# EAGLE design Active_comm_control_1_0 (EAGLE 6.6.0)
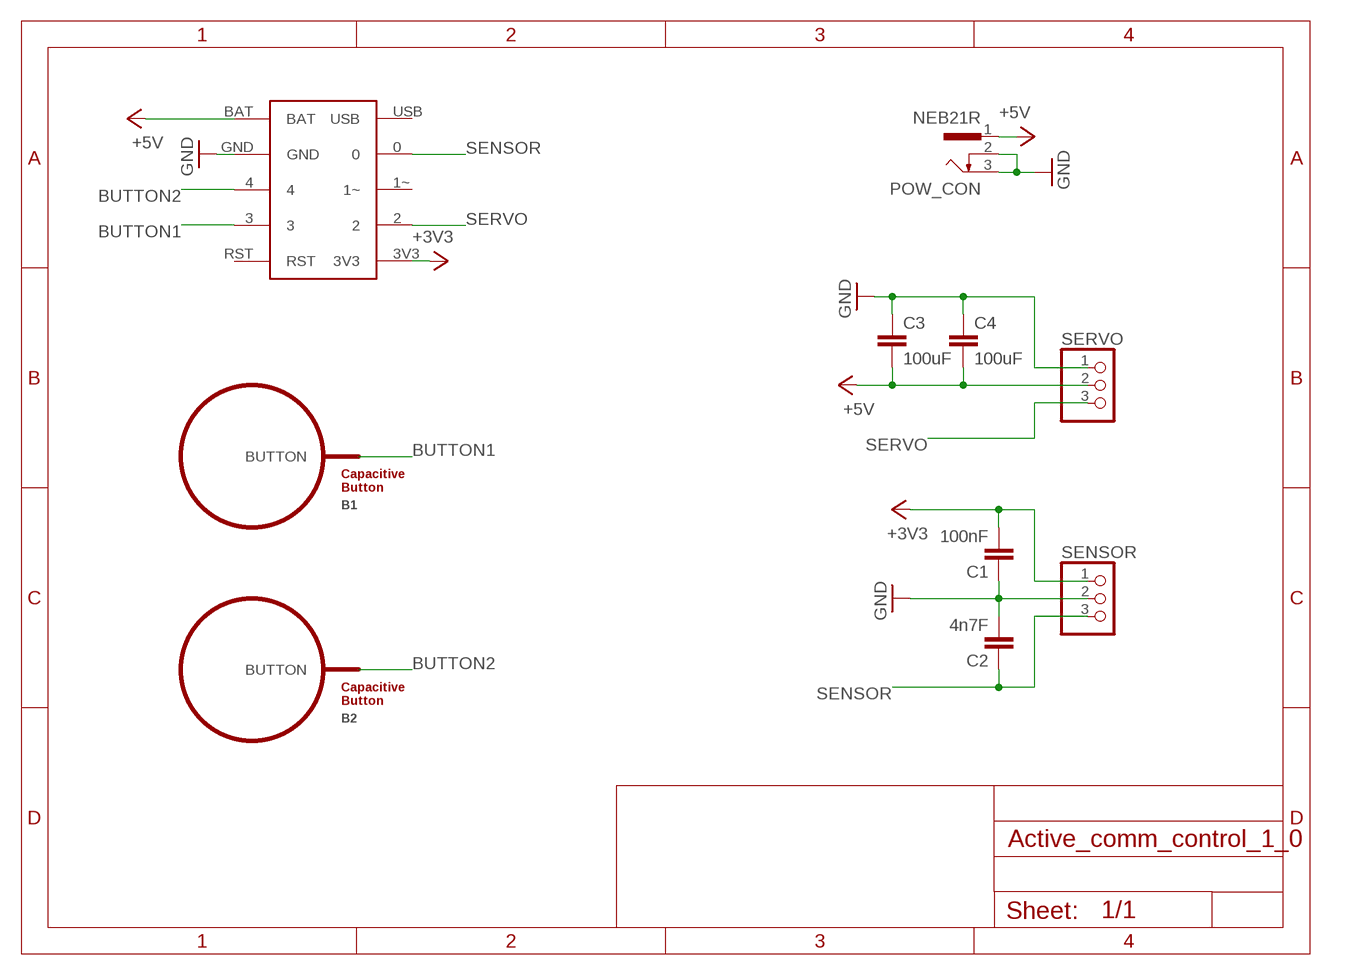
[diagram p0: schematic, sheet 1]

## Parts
B1  BUTTON_PASSIVE10MM  [BUTTON_PASSIVE_10MM]
B2  BUTTON_PASSIVE10MM  [BUTTON_PASSIVE_10MM]
C1  100nF  C-EUC0805  [C0805]
C2  4n7F  C-EUC0805  [C0805]
C3  100uF  C-EUC1206  [C1206]
C4  100uF  C-EUC1206  [C1206]
POW_CON  NEB21R  [NEB21R]
SENSOR  PINHD-1X3  [1X03]
SERVO  PINHD-1X3  [1X03]
TRINKET-M0  TRINKET-M0  [TRINKET-M0-NO-HOLES]

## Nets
+3V3: C1.2 SENSOR.1 TRINKET-M0.3V3
+5V: C3.2 C4.2 POW_CON.1 SERVO.2 TRINKET-M0.BAT
BUTTON1: B1.BUTTON TRINKET-M0.3
BUTTON2: B2.BUTTON TRINKET-M0.4
GND: C1.1 C2.2 C3.1 C4.1 POW_CON.2 POW_CON.3 SENSOR.2 SERVO.1 TRINKET-M0.GND
SENSOR: C2.1 SENSOR.3 TRINKET-M0.0
SERVO: SERVO.3 TRINKET-M0.2
Unconnected: TRINKET-M0.1~ TRINKET-M0.RST TRINKET-M0.USB

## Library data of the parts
B1 B2 = TouchWidgets:BUTTON_PASSIVE: Button, Passive Capacitive/Touch Sensing Type
C1 C2 = resistor:C-EU: CAPACITOR, European symbol
C3 C4 = rcl:C-EU: CAPACITOR, European symbol
POW_CON = con-lumberg:NEB21R: Netzgeräte-Einbaukupplung abgewinkelte Ausführung mit Öffner Source: http://www.lumberg.com/Produkte/PDFs/NEB21R.pdf; MPN: NEB 21 R; OC_FARNELL: 1217037; OC_NEWARK: 97K6458
SENSOR SERVO = adafruit:PINHD-1X3: PIN HEADER
TRINKET-M0 = adafruit:TRINKET-M0

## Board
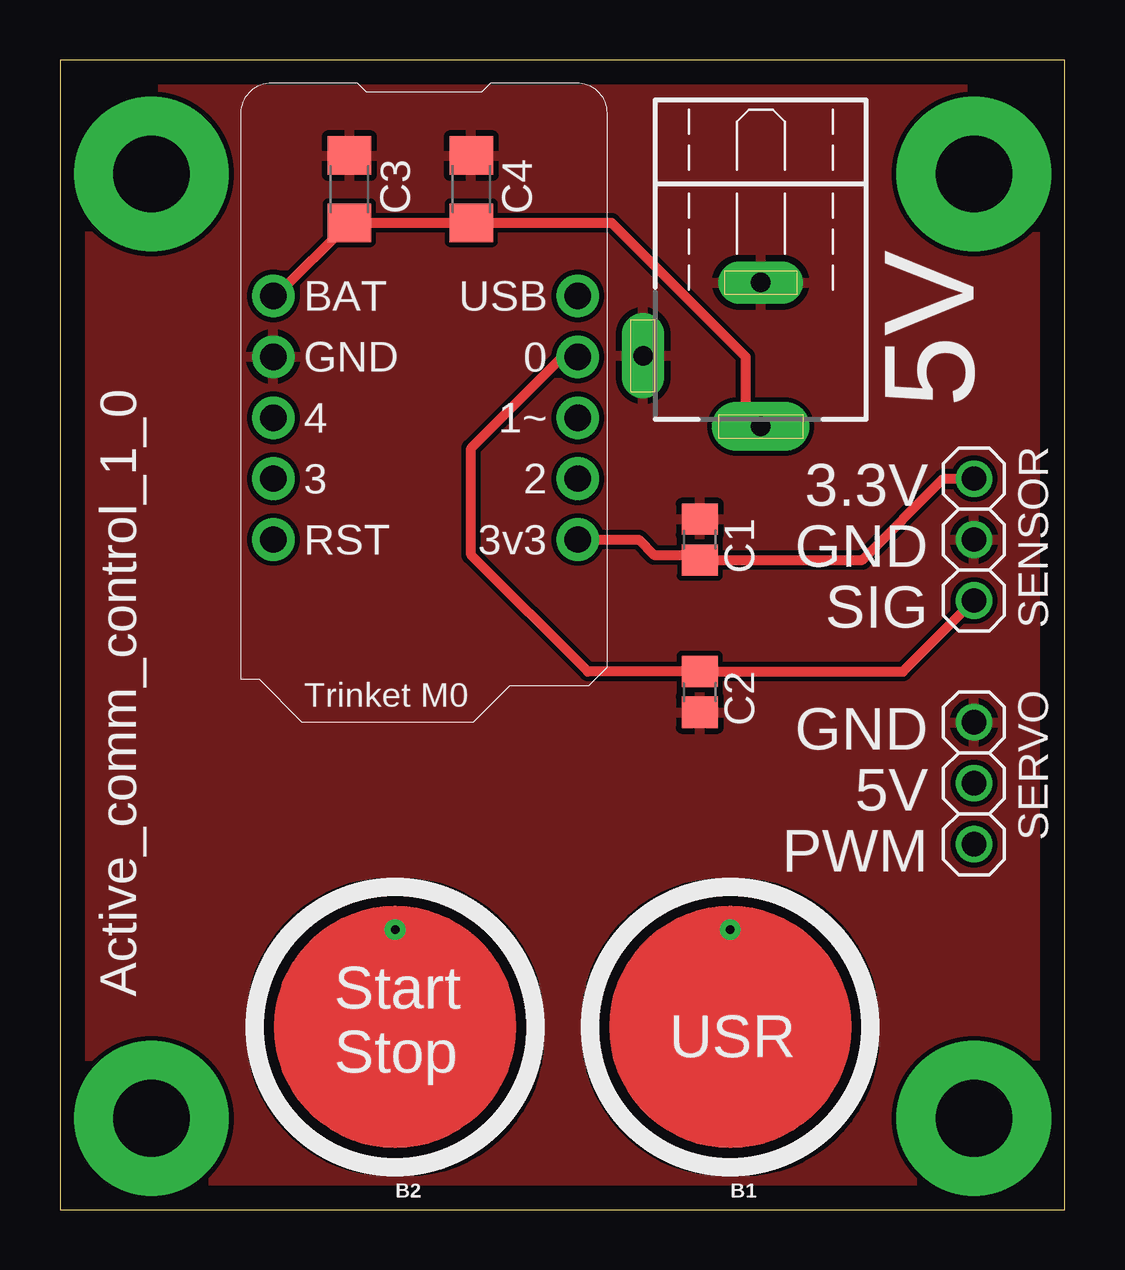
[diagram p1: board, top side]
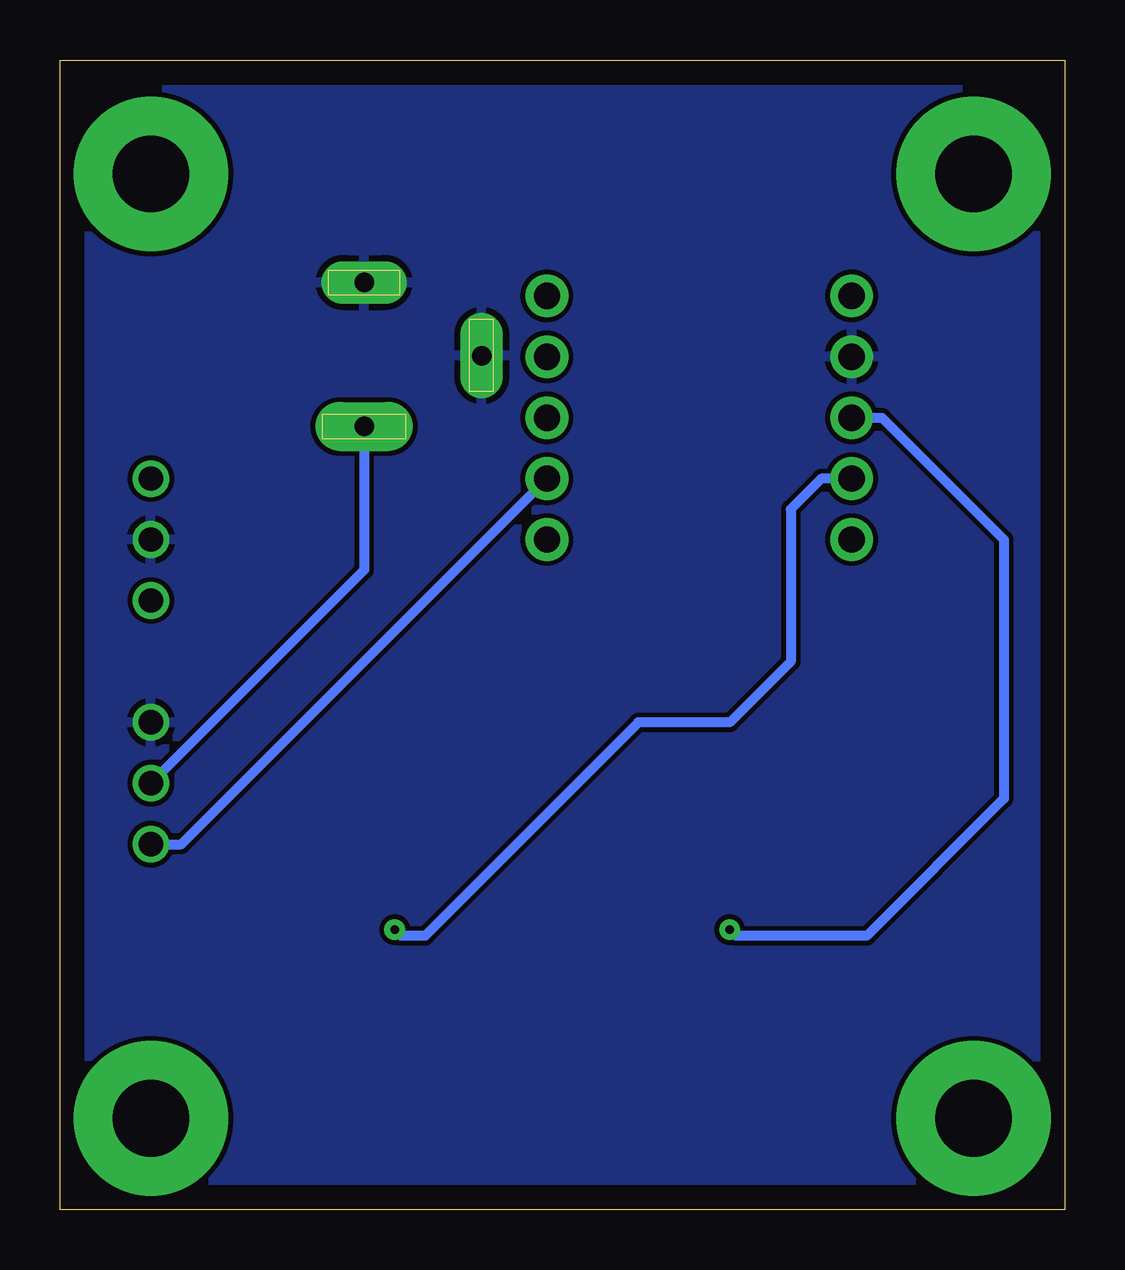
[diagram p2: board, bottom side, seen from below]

Size 41.89 x 47.93 mm. Coordinates in mm from the lower left corner, seen from the top.
Outline: 0,0 41.89,0 41.89,47.93 0,47.93 0,0
Copper layers (1*16): Top 0.035mm / dielectric 1.5mm / Bottom 0.035mm
Design rules "default": minimum track width 10mil, minimum drill 24mil, track to track 8mil, track to pad 8mil, pad to pad 8mil, via to via 8mil, smd to smd 8mil, copper to edge 40mil, drill to drill 8mil, minimum pad ring 10mil, minimum via ring 8mil, stop-mask expansion 4mil, vias tented up to drill 0mil, thermal gap 10mil

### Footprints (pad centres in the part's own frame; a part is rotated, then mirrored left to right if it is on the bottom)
BUTTON_PASSIVE_10MM = drill 0.356: BUTTON 0,4.064
C0805 = smd 1.3 x 1.5: 1 -0.85,0; 2 0.85,0
C1206 = smd 1.6 x 1.8: 1 -1.4,0; 2 1.4,0
NEB21R = drill 0.813 pad 2.032 long: 1 0,7.35 | drill 0.813 pad 1.778 long: 2 4.9,4.4; 3 0,1.35
1X03 = drill 1.016: 1 -2.54,0; 2 0,0; 3 2.54,0
TRINKET-M0-NO-HOLES = drill 1.1 pad 1.778: 0 6.35,2.54; 1~ 6.35,0; 2 6.35,-2.54; 3 -6.35,-2.54; 3V3 6.35,-5.08; 4 -6.35,0; BAT -6.35,5.08; GND -6.35,2.54; RST -6.35,-5.08; USB 6.35,5.08

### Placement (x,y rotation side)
B1  27.94,7.62 0 top
B2  13.97,7.62 0 top
C1  26.67,27.94 270 top
C2  26.67,21.59 270 top
C3  12.06,42.55 270 top
C4  17.14,42.55 270 top
POW_CON  29.21,40.01 180 top
SENSOR  38.1,27.94 270 top
SERVO  38.1,17.78 270 top
TRINKET-M0  15.24,33.02 0 top

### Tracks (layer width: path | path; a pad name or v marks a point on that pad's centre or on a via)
+3V3
  Top 0.406: TRINKET-M0.3V3 24.13,27.94 24.77,27.3 26.45,27.3 C1.2 33.44,27.09 36.83,30.48 SENSOR.1
+5V
  Top 0.406: TRINKET-M0.BAT 9.02,38.1 C3.2 C4.2 22.99,41.15 28.57,35.56 28.57,33.29 POW_CON.1
  Bottom 0.406: POW_CON.1 29.21,26.67 SERVO.2
BUTTON1
  Bottom 0.406: TRINKET-M0.3 10.16,30.48 11.43,29.21 11.43,22.86 13.97,20.32 17.78,20.32 26.67,11.43 27.69,11.43 B1.BUTTON
BUTTON2
  Bottom 0.406: TRINKET-M0.4 7.62,33.02 2.54,27.94 2.54,17.14 8.26,11.43 13.72,11.43 B2.BUTTON
GND
  pour Bottom: 0,48.26 0,0 41.91,0 41.91,48.26
  pour Top: 0,48.26 0,0 41.91,0 41.91,48.26
N$1  (via drill 3.2 pad 6.45)
  other vias: 38.1,3.81
N$2  (via drill 3.2 pad 6.45)
  other vias: 38.1,43.18
N$3  (via drill 3.2 pad 6.45)
  other vias: 3.81,43.18
N$4  (via drill 3.2 pad 6.45)
  other vias: 3.81,3.81
SENSOR
  Top 0.406: SENSOR.3 35.14,22.44 C2.1 22.01,22.44 17.14,27.3 17.14,31.75 20.95,35.56 TRINKET-M0.0
SERVO
  Bottom 0.406: SERVO.3 36.83,15.24 TRINKET-M0.2

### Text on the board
tPlace: 5V | 3.3V | GND | SIG | GND | 5V | PWM | Active_comm_control_1_0 | Start / Stop | USR

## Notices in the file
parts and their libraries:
TouchWidgets: License : http://creativecommons.org/licenses/by-sa/4.0/ (Creative Commons 4.0)
TouchWidgets: License : http://creativecommons.org/licenses/by-sa/3.1/ (Creative Commons 3.1)
